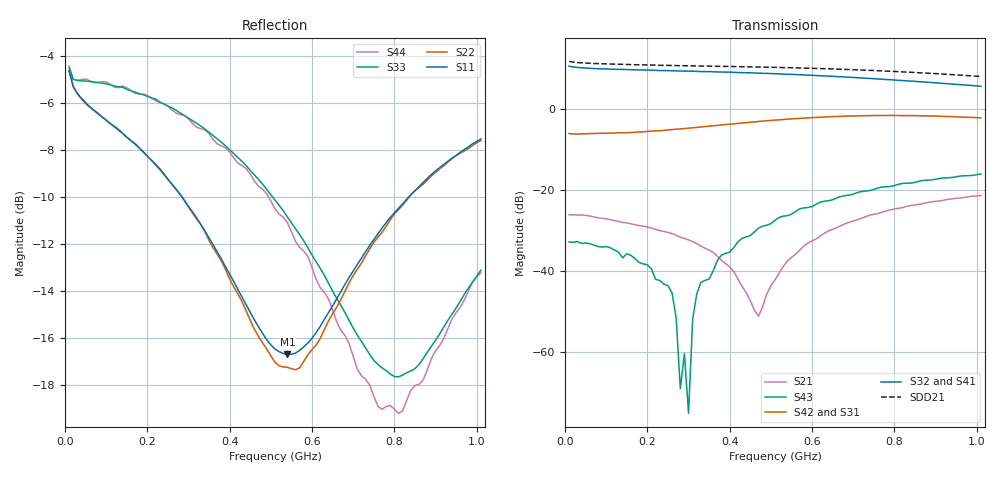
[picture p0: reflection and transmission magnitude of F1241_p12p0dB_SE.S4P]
! Integrated Device Technology
! Corporate Headquarters
! 6024 Silver Creek Valley Road
! San Jose, CA 95138  USA
! Phone:  1-408-284-8200
! Toll Free:  1-800-223-1366
! Webpage:  http://www.idt.com/
! Timing and RF Division
! 515 Groton Road, Suite 102
! Westford, MA 01886-6024
! Device:  F1241
! Description: Dual Intermediate Frequency Digital Variable Gain Amplifier
! Frequency:  10.0 -  500.00 MHz
! Package:  5x5 mm QFN Plastic Package: 32 pin
! Ports:  8 RF, 20 DC
!  Pin  1  = GA3  Pin 17  = RF OUT_B+
!  Pin  2  = GA4  Pin 18  = RF OUT_B-
!  Pin  3  = GA5  Pin 19  = STBY_B
!  Pin  4  = ISET_A  Pin 20  = Ground
!  Pin  5  = ISET_B  Pin 21  = Ground
!  Pin  6  = GB5  Pin 22  = STB_A
!  Pin  7  = GB4  Pin 23  = RF OUT_A-  = Port 4
!  Pin  8  = GB3  Pin 24  = RF OUT_A+  = Port 3
!  Pin  9  = GB2  Pin 25  = NO CONNECT
!  Pin 10  = GB1  Pin 26  = NO CONNECT
!  Pin 11  = RF IN_B+  Pin 27  = VCC
!  Pin 12  = RF IN_B-  Pin 28  = Ground
!  Pin 13  = Ground  Pin 29  = RF IN_A-  = Port 2
!  Pin 14  = VCC  Pin 30  = RF IN_A+  = Port 1
!  Pin 15  = NO CONNECT  Pin 31  = GA1
!  Pin 16  = NO CONNECT  Pin 32  = GA2
! State:  8
! Gain State:  12.0 dB
! Voltages:  Vcc = +5.00 Volts  Icc approximately 160.0 mA or 80 mA per channel.
! Data:  The device was measured on a custom evaluation board which has
!  individual transmission lines to the RF pins.  Data was collected
!  using a calibrated network analyzer.  The evaluation board was
!  de-embedded using a port reference technique.
!  The reference plane is the edge of the package pin.
!  Only Channel A was measured.
!  This data is in single-ended operation.  If your needs are balanced
!  or differential S-parameters then this file needs to be used a
!  linear simulator.
! Misc:  Lot Code  160028MY
!  Action Tracker AT004
! Date Measured:  2014-08-14
! Date:  2014-08-28  MJV
! Note:
!  Integrated Device Technology supplies this data as a sample of measured
!  data at the package pin for this product.  Your particular data for this
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# Hz S dB R 50
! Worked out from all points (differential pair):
!   101 points, 10 MHz to 1.01 GHz, reference 50 ohm
!   strongest paths, dB at 10 MHz, 260 MHz, 510 MHz, 760 MHz, 1.01 GHz:
!     S32: 10.7, 9.6, 8.9, 7.6, 5.7
!     S41: 10.7, 9.5, 8.7, 7.4, 5.5
!     S42: -5.9, -5.0, -2.6, -1.5, -2.1
!     S31: -6.0, -5.1, -2.8, -1.7, -2.2
!     S43: -32.8, -45.5, -27.5, -19.5, -16.0
!     S21: -26.1, -30.8, -42.2, -25.8, -21.3
!   taken as a pair (ports 2,1 in; 3,4 out), SDD21 dB: 11.9, 10.9, 10.4, 9.6, 8.2
!   lowest |S11| = -16.7 dB at 540 MHz (marker M1), VSWR 1.34, Z = 39.6 - j8.09 ohm
!   |S11| at or under -10 dB: 283.8 MHz to 834.8 MHz (550.9 MHz wide, 98.5 % of centre)
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1e7  -4.61 -15.7  -26.08 6.1  -49.71 44.5  -19.87 10.5
     -26.08 6.0  -4.61 -15.6  -19.89 10.2  -49.49 43.3
     -5.96 1.3  10.73 -177.9  -4.50 -13.1  -32.84 28.4
     10.75 -177.8  -5.95 1.4  -32.81 27.6  -4.42 -13.3
2.5e8  -9.24 -45.3  -30.51 -27.3  -32.31 54.0  -20.24 -11.0
       -30.46 -31.4  -9.24 -43.1  -20.20 -11.2  -32.34 53.3
       -5.18 -6.7  9.63 144.5  -6.12 -23.4  -42.00 -51.7
       9.58 143.8  -5.08 -6.9  -43.65 -28.1  -6.12 -22.6
3e8  -10.40 -54.3  -32.09 -30.0  -30.88 49.7  -20.11 -13.1
     -32.32 -34.9  -10.42 -52.0  -20.06 -13.3  -30.86 49.0
     -4.75 -9.0  9.50 138.1  -6.64 -28.0  -47.53 -110.6
     9.44 137.4  -4.62 -9.3  -75.26 128.4  -6.67 -27.2
3.3e8  -11.18 -60.3  -33.32 -29.1  -30.14 46.7  -20.00 -14.9
       -33.86 -37.7  -11.17 -57.4  -19.95 -14.7  -30.12 45.8
       -4.52 -10.7  9.40 134.2  -6.97 -30.9  -44.63 -146.6
       9.35 133.4  -4.34 -11.1  -42.86 140.2  -7.08 -29.1
4.7e8  -15.54 -102.3  -42.60 24.3  -27.54 33.2  -19.55 -23.2
       -51.24 37.6  -15.94 -98.7  -19.41 -22.9  -27.51 31.8
       -3.18 -21.5  9.00 115.9  -9.25 -46.2  -31.21 142.3
       8.90 115.1  -2.98 -22.9  -29.37 125.4  -9.54 -43.9
5.4e8  -16.71 -136.9  -37.82 72.4  -26.66 26.5  -19.36 -28.0
       -37.55 95.6  -17.26 -134.8  -19.19 -28.0  -26.57 24.5
       -2.60 -28.7  8.73 106.9  -10.84 -56.0  -27.08 129.7
       8.61 105.9  -2.41 -30.5  -26.30 113.8  -11.09 -53.5
1.01e9  -7.52 120.4  -21.94 52.5  -23.97 -14.4  -20.13 -64.4
        -21.32 54.1  -7.59 120.2  -19.61 -65.0  -23.89 -18.6
        -2.24 -88.2  5.75 50.3  -13.12 164.7  -16.70 60.4
        5.54 49.7  -2.09 -91.6  -15.98 54.1  -13.23 157.5
